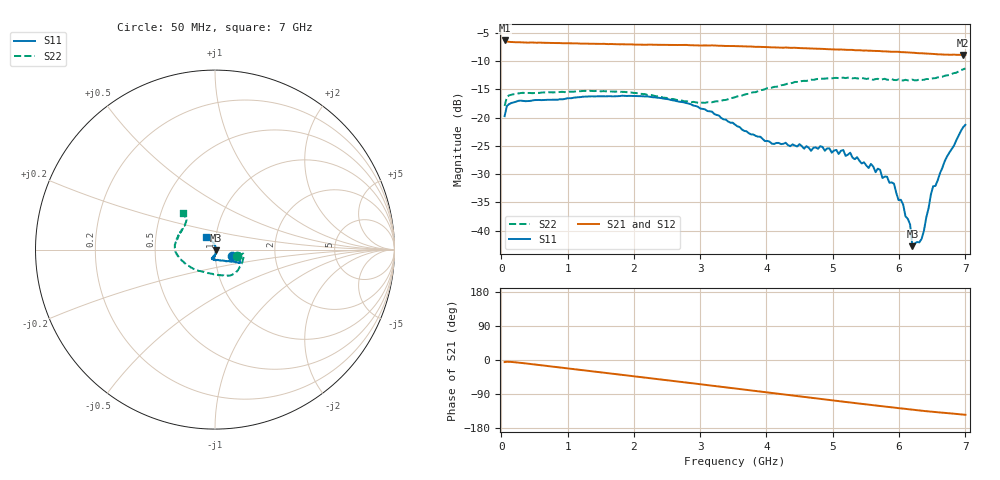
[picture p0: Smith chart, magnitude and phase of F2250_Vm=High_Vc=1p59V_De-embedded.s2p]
! Integrated Device Technology
! Corporate Headquarters
! 6024 Silver Creek Valley Road
! San Jose, CA 95138  USA
! Phone:  1-408-284-8200
! Toll Free:  1-800-223-1366
! Webpage:  http://www.idt.com/
! Timing and RF Division
! 515 Groton Road, Suite 102
! Westford, MA 01886-6024
! Device:  F2250
! Description: Voltage Variable RF Attenuator
! Frequency:  50.0 -  6000.00 MHz
! Package:  3x3 mm Thin QFN Plastic Package: 16 pin
! Ports:  2 RF, 3 DC
!  Pin  1  = GND
!  Pin  2  = NC
!  Pin  3  = RF1  = Port 1
!  Pin  4  = NC
!  Pin  5  = GND
!  Pin  6  = GND
!  Pin  7  = GND
!  Pin  8  = GND
!  Pin  9  = NC
!  Pin 10  = RF2  = Port 2
!  Pin 11  = NC
!  Pin 12  = GND
!  Pin 13  = GND
!  Pin 14  = VCNTRL
!  Pin 15  = VDD
!  Pin 16  = VMODE
! Vcntrl:  1.590 Volts
! Vmode:  +3.300 Volts
! Vdd:  +3.30  Volts
! Current:  1.330 mA
! Data:  The device was measured on a the F2250 evaluation board which has
!  individual transmission lines to the RF pins.  Data was collected
!  using a calibrated network analyzer.  The evaluation board was
!  de-embedded using a TRL calibration technique.
!  The reference plane is the edge of the package pin.
! Misc:  SN 10
!  Action Tracker AT0258
! Date Measured:  2014-11-26
! Date:  2015-10-15  MJV
! Note:
!  Integrated Device Technology supplies this data as a sample of measured
!  data at the package pin for this product.  Your particular data for this
!  product may vary.
!  Data was taken at 25 degrees C.
!  Integrated Device Technology reserves the right to change this data at anytime.
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# GHz S dB R 50
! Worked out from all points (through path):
!   201 points, 50 MHz to 7 GHz, reference 50 ohm
!   highest |S21| = -6.34 dB at 50 MHz (marker M1); lowest = -8.9 dB at 6.965 GHz (marker M2)
!   group delay of S21, straight-line fit = 57.9 ps
!   lowest |S11| = -42.8 dB at 6.201 GHz (marker M3), VSWR 1.01, Z = 50.6 - j0.461 ohm
!   |S11| at or under -10 dB: start of sweep to end of sweep
!   |S22| runs from -17.9 to -11.3 dB; largest |S21 - S12| = 0.0024
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0.05  -19.74 -20.5  -6.34 -5.5  -6.34 -5.4  -17.93 -15.9
0.08475  -17.93 -10.4  -6.53 -4.6  -6.54 -4.6  -16.33 -9.3
0.2585  -17.02 -8.4  -6.65 -6.9  -6.67 -6.9  -15.72 -12.0
1.2315  -16.29 -24.7  -6.90 -27.1  -6.91 -27.1  -15.28 -42.7
2.37825  -16.49 -29.2  -7.11 -50.7  -7.12 -50.7  -16.21 -70.8
2.969  -18.09 -32.1  -7.22 -63.3  -7.20 -63.3  -17.37 -97.4
3.525  -21.24 -46.7  -7.33 -75.3  -7.34 -75.4  -16.39 -130.4
4.081  -24.61 -75.9  -7.56 -87.3  -7.56 -87.3  -14.70 -156.0
4.7065  -25.35 -106.0  -7.78 -100.6  -7.78 -100.6  -13.31 -174.3
5.2625  -26.21 -103.9  -8.01 -112.1  -8.00 -112.2  -12.94 172.6
5.71425  -29.25 -90.1  -8.22 -121.4  -8.23 -121.4  -13.29 160.9
5.85325  -31.52 -84.8  -8.31 -124.1  -8.32 -124.2  -13.30 156.4
5.92275  -31.69 -82.3  -8.34 -125.5  -8.33 -125.6  -13.34 155.7
5.99225  -34.60 -82.3  -8.35 -127.1  -8.37 -127.2  -13.23 153.2
6.06175  -35.40 -64.5  -8.41 -128.3  -8.40 -128.4  -13.43 150.4
6.0965  -37.47 -64.6  -8.44 -129.1  -8.44 -129.2  -13.30 149.7
6.166  -38.91 -45.8  -8.48 -130.4  -8.51 -130.4  -13.40 147.0
6.20075  -42.75 -38.7  -8.50 -131.2  -8.52 -131.2  -13.27 146.4
6.33975  -41.46 55.5  -8.61 -133.7  -8.58 -133.9  -13.33 141.8
6.5135  -32.15 95.0  -8.71 -136.8  -8.73 -137.0  -13.04 136.5
6.96525  -21.71 122.7  -8.90 -144.0  -8.90 -144.1  -11.47 132.0
7  -21.27 123.6  -8.90 -144.5  -8.91 -144.6  -11.29 131.2
